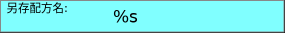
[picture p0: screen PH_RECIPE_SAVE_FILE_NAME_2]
VISUALIZATION PH_RECIPE_SAVE_FILE_NAME_2  // 285x33
VAR_IN_OUT
	RECIPE_CTRL_V2 : ST_RecipeCtrl_2;
END_VAR
VAR_INPUT
	Right_Edge_Rel : UDINT;
END_VAR
    Rectangle (0,0 285x33), "另存配方名:", input disabled if: true, text list: 'TextList_Recipe', text index: 102
        p874137650: Right_Edge_Rel
    Rectangle (110,0 175x33), "%s", text variable: RECIPE_CTRL_V2.sgFileNameSave
        p874137650: Right_Edge_Rel
        OnMouseClick: write the text variable via Edit
END_VISUALIZATION
